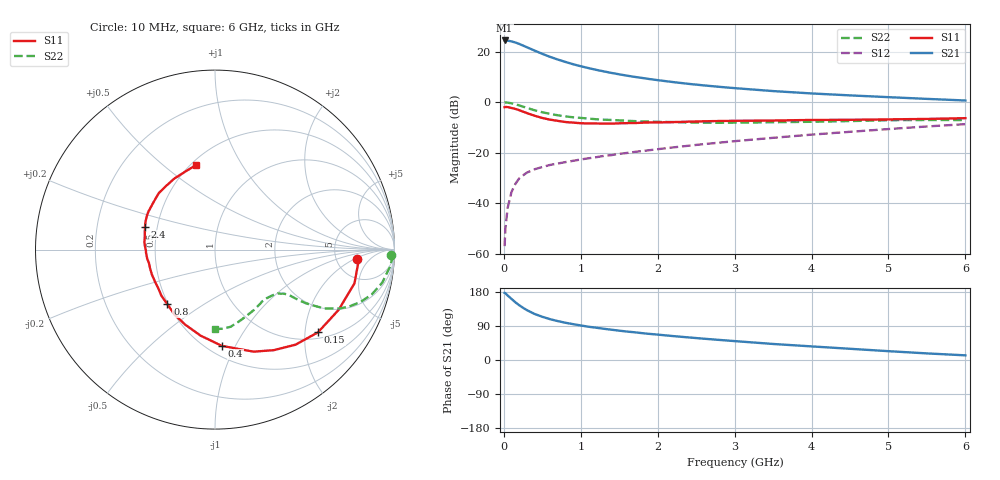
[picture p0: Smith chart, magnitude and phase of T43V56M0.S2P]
! Infineon Technologies  Discrete & RF Semiconductors
! BFR182T
! Si NPN RF Bipolar Junction Transistor in SC75
! VCE = 3.5 V  IC = 6 mA
! Common Emitter S-Parameters:  October  1999
# GHz  S  MA  R  50
!  f  S11  S21  S12  S22
! GHz  MAG  ANG  MAG  ANG  MAG  ANG  MAG  ANG
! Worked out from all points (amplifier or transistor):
!   36 points, 10 MHz to 6 GHz, reference 50 ohm
!   highest |S21| = 24.5 dB at 10 MHz (marker M1)
!   |S21| within 3 dB of that: start of sweep to 323.1 MHz
!   unconditionally stable (mu >= 1): 1.315 GHz to 3.945 GHz
!   at 250 MHz: K = 0.31, MSG = 25.7 dB, |S12| = -29.0 dB
!   at 1.4 GHz: K = 1.03, MAG = 15.2 dB, |S12| = -21.0 dB
!   at 6 GHz: K = 0.84, MSG = 4.7 dB, |S12| = -8.7 dB
!   lowest NFmin = 1.25 dB at 450 MHz
!   S11 on the Smith chart (normalised r, x): 10 MHz: 8.07, -2.31; 150 MHz: 1.16, -2.34; 400 MHz: 0.59, -0.88; 800 MHz: 0.49, -0.36; 2.4 GHz: 0.43, +0.13; 6 GHz: 0.53, +0.65
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0.01  0.7947 -3.8  16.71 177.1  0.0014 80.8  0.981 -1.9
0.02  0.803 -4.2  16.66 176.2  0.0031 94.8  0.9912 -2.4
0.05  0.7995 -13.6  16.6 170.1  0.0081 88.1  0.9785 -5.8
0.1  0.7666 -25.9  15.98 161.2  0.0167 77.8  0.9497 -11.2
0.15  0.736 -38.8  15.23 152.2  0.024 71.6  0.909 -15.9
0.2  0.6943 -49.7  14.29 144.5  0.0309 67.4  0.863 -19.7
0.25  0.6489 -59.7  13.24 137.7  0.0354 63.8  0.8143 -22.8
0.3  0.6079 -69.3  12.26 131.6  0.0402 61.7  0.7706 -25.2
0.4  0.5378 -85.9  10.52 121.5  0.0468 56.9  0.6908 -28.3
0.5  0.486 -99.5  9.077 114.0  0.0519 54.8  0.6314 -29.6
0.6  0.45 -111.6  7.912 107.8  0.057 54.6  0.5861 -30.6
0.7  0.4268 -121.8  7.011 102.7  0.0608 54.4  0.5504 -31.0
0.8  0.4039 -131.1  6.277 98.3  0.0648 54.2  0.5234 -31.3
1.1  0.3786 -152.9  4.738 87.8  0.0772 56.2  0.4722 -32.1
1.4  0.3753 -168.3  3.796 79.9  0.0893 58.3  0.4435 -33.7
1.6  0.3843 -177.0  3.353 75.1  0.0985 59.4  0.4274 -34.8
2.2  0.4027 166.1  2.502 63.1  0.1269 62.0  0.4026 -40.6
2.4  0.4108 161.8  2.309 59.6  0.1369 62.5  0.3957 -43.0
3.5  0.4328 142.1  1.659 42.3  0.1966 62.1  0.4002 -57.2
4.5  0.4471 127.8  1.363 29.6  0.2586 59.0  0.4221 -71.5
5.5  0.4653 110.7  1.162 17.4  0.3298 54.2  0.4432 -84.4
6  0.4821 102.7  1.079 12.3  0.3669 50.8  0.4423 -89.9
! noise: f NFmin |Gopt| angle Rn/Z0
0.45  1.25  0.25  39  0.3
0.9  1.4  0.25  78  0.23
1.8  1.95  0.21  151  0.2
